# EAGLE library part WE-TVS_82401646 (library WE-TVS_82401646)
TVS Diode Array WE-TVS, Super Speed Serie - Low capazity - No leakage current - Low clamping voltage - high ESD voltage protection -- USB 3.0
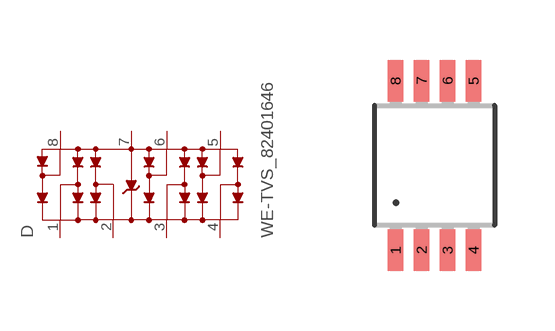
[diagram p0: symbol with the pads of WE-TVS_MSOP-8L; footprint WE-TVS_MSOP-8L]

Designator prefix D

## WE-TVS_82401646 (MPN: 82401646; OC_FARNELL: 1825864; OC_NEWARK: 79R6953; PACKAGE: MSOP-8L; SUPPLIER: Wuerth Elektronik)  [WE-TVS_MSOP-8L]
1  1  pas
2  2  pas
3  3  pas
4  4  pas
5  5  pas
6  6  pas
7  GND  pwr
8  VDD  pwr

## Footprint WE-TVS_MSOP-8L (pad centres in mm)
TVS Diode Array WE-TVS
smd 0.38 x 1.04: 1 -0.975,-2.12; 2 -0.325,-2.12; 3 0.325,-2.12; 4 0.975,-2.12; 5 0.975,2.12; 6 0.325,2.12; 7 -0.325,2.12; 8 -0.975,2.12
